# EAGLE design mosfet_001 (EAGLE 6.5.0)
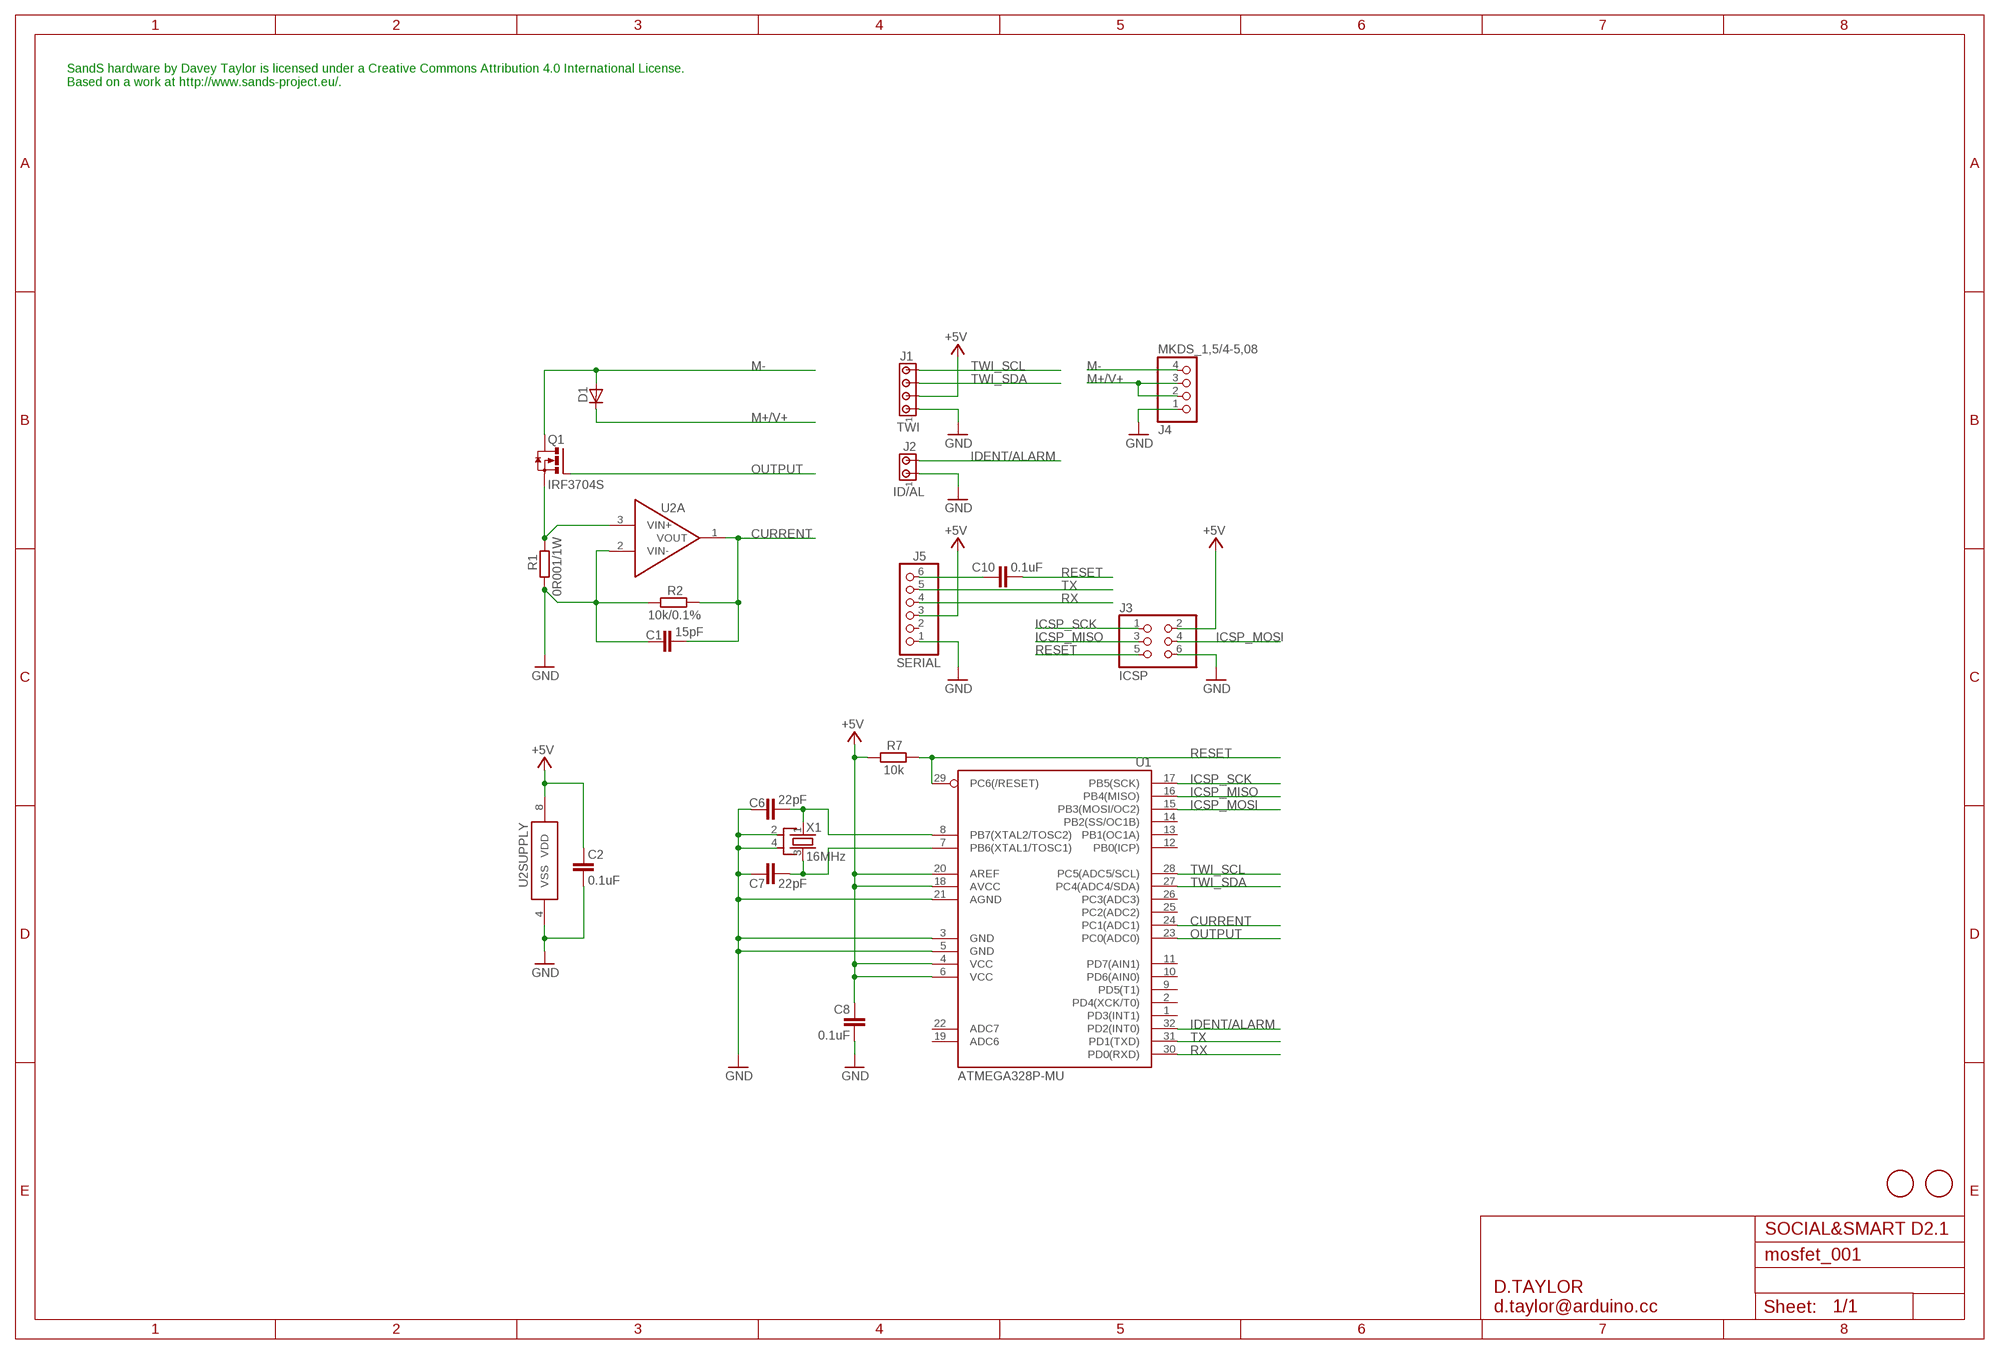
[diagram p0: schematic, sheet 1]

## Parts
C1  15pF  C-EUC0603  [C0603]
C2  0.1uF  C-EUC0603  [C0603]
C6  22pF  C-EUC0603  [C0603]
C7  22pF  C-EUC0603  [C0603]
C8  0.1uF  C-EUC0603  [C0603]
C10  0.1uF  C-EUC0603  [C0603]
D1  DIODE-SMB  [SMB]
J1  TWI  MTA04-100  [10X04MTA]
J2  ID/AL  MTA02-100  [10X02MTA]
J3  ICSP  PINHD-2X3  [2X03]
J4  MKDS_1,5/4-5,08  [MKDS1,5/4-5,08]
J5  SERIAL  PINHD-1X6  [1X06]
Q1  IRF3704S  [D2PACK]
R1  0R001/1W  R-EU_R2512  [R2512]
R2  10k/0.1%  R-EU_R0603  [R0603]
R7  10k  R-EU_R0603  [R0603]
U1  ATMEGA328P-MU  [MLF32-M1-A]
U2  LTC6081  [MSOP08]
U$5  FIDUCIALMOUNT  [FIDUCIA-MOUNT]
U$6  FIDUCIALMOUNT  [FIDUCIA-MOUNT]
X1  16MHz  CRYSTAL-KX7  [XTAL-3.2-2.5]

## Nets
+5V: C2.1 C8.1 J1.2 J3.2 J5.3 R7.1 U1.4(VCC) U1.6(VCC) U1.18(AVCC) U1.20(AREF) U2.8(SUPPLY:VDD)
CURRENT: C1.2 R2.2 U1.24(PC1(ADC1)) U2.1(A:VOUT)
GND: C1.1 C2.2 C6.1 C7.1 C8.2 J1.1 J2.1 J3.6 J4.1 J5.1 R1.1 R2.1 U1.3(GND) U1.5(GND) U1.21(AGND) U2.2(A:VIN-) U2.4(SUPPLY:VSS) X1.2(SH1) X1.4(SH2)
ICSP_MISO: J3.3 U1.16(PB4(MISO))
ICSP_MOSI: J3.4 U1.15(PB3(MOSI/OC2))
ICSP_SCK: J3.1 U1.17(PB5(SCK))
IDENT/ALARM: J2.2 U1.32(PD2(INT0))
M+/V+: D1.C J4.2 J4.3
M-: D1.A J4.4 Q1.2(D)
N$1: Q1.3(S) R1.2 U2.3(A:VIN+)
N$6: C6.2 U1.8(PB7(XTAL2/TOSC2)) X1.1(X1)
N$7: C7.2 U1.7(PB6(XTAL1/TOSC1)) X1.3(X2)
N$9: C10.1 J5.6
OUTPUT: Q1.1(G) U1.23(PC0(ADC0))
RESET: C10.2 J3.5 R7.2 U1.29(PC6(/RESET))
RX: J5.4 U1.30(PD0(RXD))
TWI_SCL: J1.4 U1.28(PC5(ADC5/SCL))
TWI_SDA: J1.3 U1.27(PC4(ADC4/SDA))
TX: J5.5 U1.31(PD1(TXD))
Unconnected: J5.2 U1.1(PD3(INT1)) U1.2(PD4(XCK/T0)) U1.9(PD5(T1)) U1.10(PD6(AIN0)) U1.11(PD7(AIN1)) U1.12(PB0(ICP)) U1.13(PB1(OC1A)) U1.14(PB2(SS/OC1B)) U1.19(ADC6) U1.22(ADC7) U1.25(PC2(ADC2)) U1.26(PC3(ADC3)) U2.5(B:VIN+) U2.6(B:VIN-) U2.7(B:VOUT)

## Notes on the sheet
- SandS hardware by Davey Taylor is licensed under a Creative Commons Attribution 4.0 International License.
  Based on a work at http://www.sands-project.eu/.
- SOCIAL&SMART D2.1
- D.TAYLOR
  d.taylor@arduino.cc

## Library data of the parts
C1 C2 C6-C8 C10 = rcl:C-EU: CAPACITOR, European symbol
D1 = diode:DIODE-: DIODE
J1 = con-amp:MTA04-100: AMP connector
J2 = con-amp:MTA02-100: AMP connector
J3 = pinhead:PINHD-2X3: PIN HEADER
J4 = d_taylor:MKDS_1,5/4-5,08
J5 = pinhead:PINHD-1X6: PIN HEADER
Q1 = transistor-power:IRF3704: SMPS MOSFET HEXFET® Power MOSFET Source: http://www.irf.com/product-info/datasheets/data/irf3704.pdf
R1 R2 R7 = rcl:R-EU_: RESISTOR, European symbol
U1 = d_taylor:ATMEGA*: MICROCONTROLLER 8 Kbytes FLASH 1 kbytes SRAM 512 bytes EEPROM USART 6-channel 10 bit ADC 2-channel 8 bit ADC Source: avr.lbr
U2 = d_taylor:LTC6081
U$5 U$6 = SmartPrj:FIDUCIALMOUNT
X1 = d_taylor:CRYSTAL-KX7

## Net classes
1 PWR: width 0.406 mm, clearance 0.254 mm

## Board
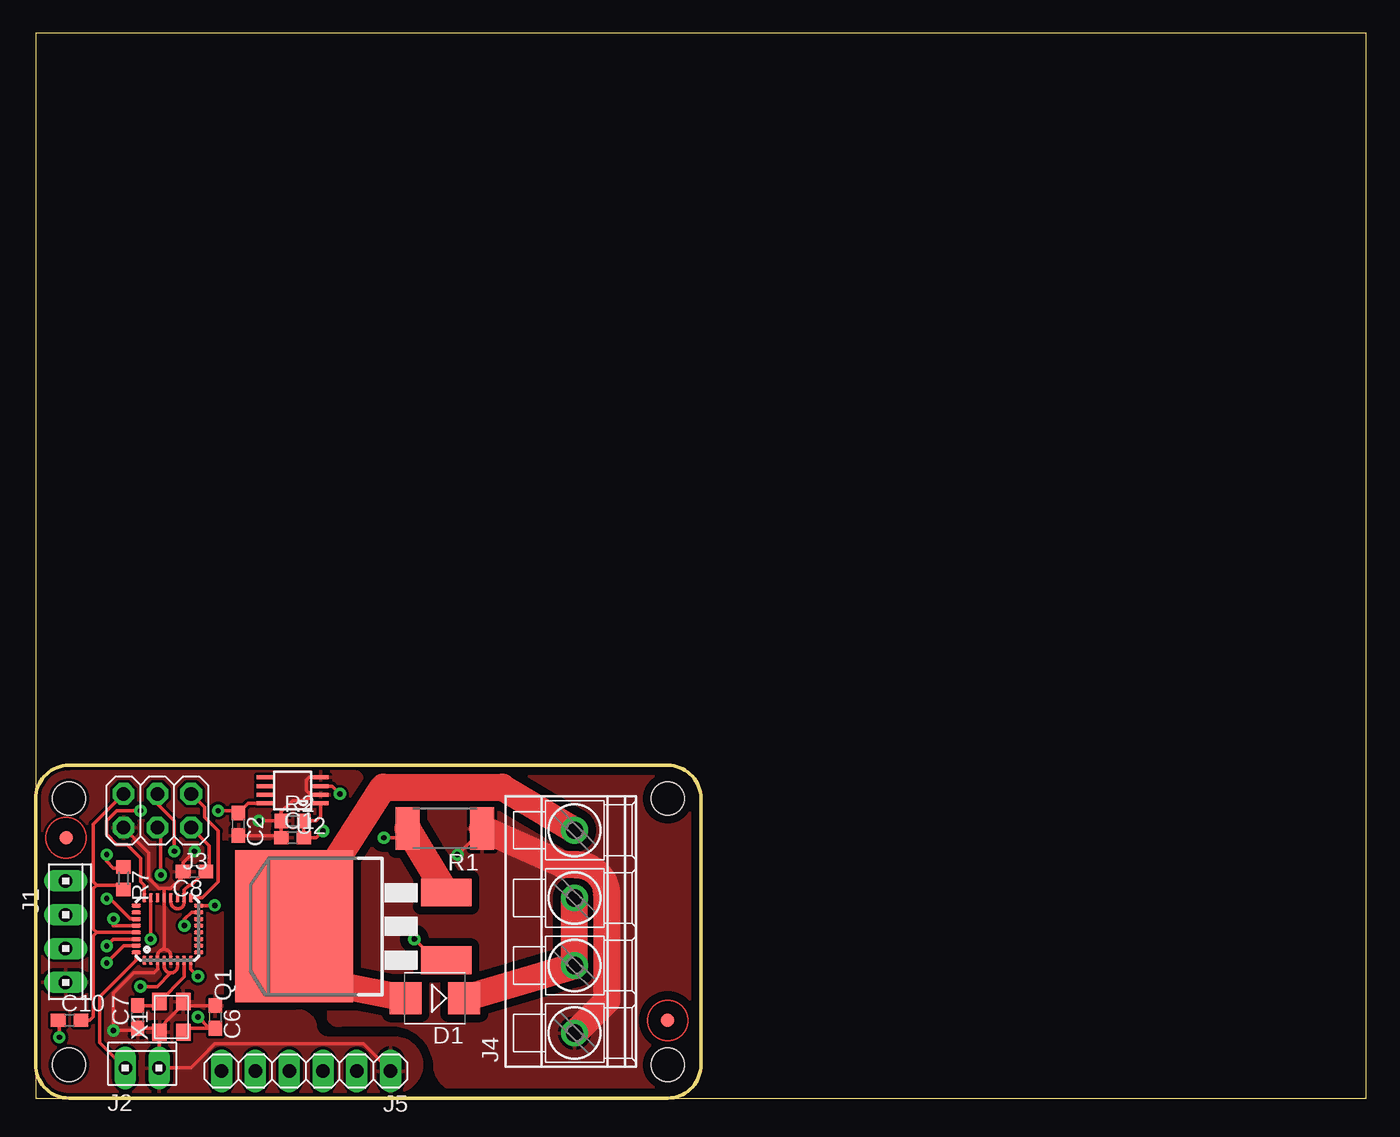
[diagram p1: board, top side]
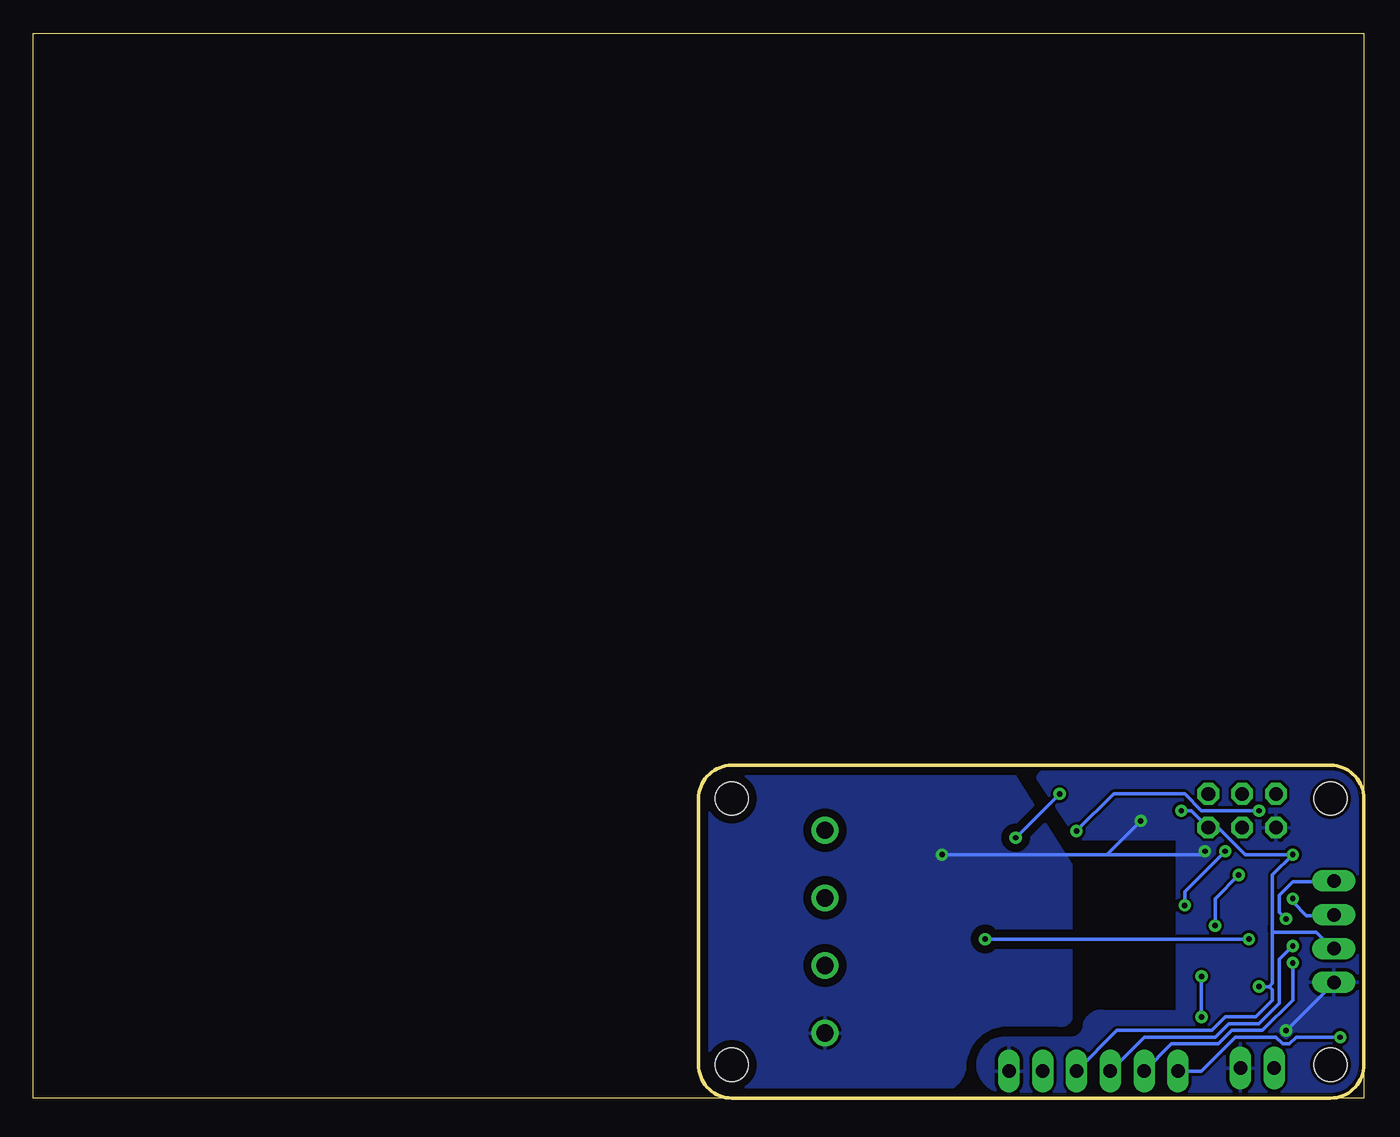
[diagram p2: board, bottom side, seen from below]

Size 100 x 80 mm. Coordinates in mm from the lower left corner, seen from the top.
Outline: 0,0 100,0 100,80 0,80 0,0
Outline: 2.5,0 47.5,0 arc90 50,2.5 50,22.5 arc90 47.5,25 2.5,25 arc90 0,22.5 0,2.5 arc90 2.5,0
Copper layers (1*16): Top 0.035mm / dielectric 1.5mm / Bottom 0.035mm
Design rules "smartprj-mini *": minimum track width 8mil, minimum drill 16mil, track to track 8mil, track to pad 8mil, pad to pad 0.200659375mm, via to via 8mil, smd to smd 4mil, copper to edge 10mil, drill to drill 8mil, minimum pad ring 12mil, minimum via ring 10mil, stop-mask expansion 2mil, vias tented up to drill 20mil, thermal gap 10mil
Holes 2.5 mm at 2.5,22.5 2.5,2.5 47.5,2.5 47.5,22.5

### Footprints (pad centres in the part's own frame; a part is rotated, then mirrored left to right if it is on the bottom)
C0603 = smd 1.1 x 1: 1 -0.85,0; 2 0.85,0
SMB = smd 2.4 x 2.4: A 2.2,0; C -2.2,0
10X04MTA = drill 1.016 long: 1 3.81,0; 2 1.27,0; 3 -1.27,0; 4 -3.81,0
10X02MTA = drill 1.016 long: 1 1.27,0; 2 -1.27,0
2X03 = drill 1.016 octagon: 1 -2.54,-1.27; 2 -2.54,1.27; 3 0,-1.27; 4 0,1.27; 5 2.54,-1.27; 6 2.54,1.27
MKDS1,5/4-5,08 = drill 1.3 pad 2: 1 -7.62,0; 2 -2.54,0; 3 2.54,0; 4 7.62,0
1X06 = drill 1.016 long: 1 -6.35,0; 2 -3.81,0; 3 -1.27,0; 4 1.27,0; 5 3.81,0; 6 6.35,0
D2PACK = smd 2.083 x 3.81: 1 -2.54,-8.89; 3 2.54,-8.89 | smd 11.43 x 8.89: 2 0,2.54
R2512 = smd 1.8 x 3.2: 1 -2.8,0; 2 2.8,0
R0603 = smd 1 x 1.1: 1 -0.85,0; 2 0.85,0
MLF32-M1-A = smd 0.7 x 0.3: 1 -2.35,1.75; 2 -2.35,1.25; 3 -2.35,0.75; 4 -2.35,0.25; 5 -2.35,-0.25; 6 -2.35,-0.75; 7 -2.35,-1.25; 8 -2.35,-1.75; 17 2.35,-1.75; 18 2.35,-1.25; 19 2.35,-0.75; 20 2.35,-0.25; 21 2.35,0.25; 22 2.35,0.75; 23 2.35,1.25; 24 2.35,1.75 | smd 0.3 x 0.7: 9 -1.75,-2.35; 10 -1.25,-2.35; 11 -0.75,-2.35; 12 -0.25,-2.35; 13 0.25,-2.35; 14 0.75,-2.35; 15 1.25,-2.35; 16 1.75,-2.35; 25 1.75,2.35; 26 1.25,2.35; 27 0.75,2.35; 28 0.25,2.35; 29 -0.25,2.35; 30 -0.75,2.35; 31 -1.25,2.35; 32 -1.75,2.35
MSOP08 = smd 0.3 x 1.2: 1 -0.976,-2.113; 2 -0.326,-2.113; 3 0.324,-2.113; 4 0.974,-2.113; 5 0.974,2.112; 6 0.324,2.112; 7 -0.326,2.112; 8 -0.976,2.112
FIDUCIA-MOUNT = smd 1.016 x 1.016: P$1 0,0
XTAL-3.2-2.5 = smd 1.3 x 1.1: 1 -1.15,-0.9; 2 1.15,-0.9; 3 1.15,0.9; 4 -1.15,0.9

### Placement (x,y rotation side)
C1  19.3,19.56 0 top
C2  15.24,20.57 270 top
C6  13.5,6.1 270 top
C7  7.66,6.1 90 top
C8  11.94,17.02 180 top
C10  2.54,5.84 0 top
D1  30,7.5 180 top
J1  2.25,12.5 270 top
J2  8,2.25 0 top
J3  9.14,21.59 180 top
J4  40.5,12.5 90 top
J5  20.32,2.03 180 top
Q1  21.96,12.9 90 top
R1  30.75,20.25 180 top
R2  19.3,20.83 0 top
R7  6.6,16.51 270 top
U1  9.91,12.7 90 top
U2  19.3,23.11 90 top
U$5  2.29,19.56 0 top
U$6  47.5,5.84 0 top
X1  10.2,6.1 90 top

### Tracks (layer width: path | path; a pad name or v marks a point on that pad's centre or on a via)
+5V  (via drill 0.41)
  Top 0.254: 11.18,15.32 U1.18 | 11.18,15.05 U1.18 | U1.4 9.66,9.9 arc90 10.16,9.4 | 10.16,9.4 arc90 10.66,9.89 U1.6 | 10.16,9.4 9.14,8.38 v7.87,8.38 | U1.18 11.16,15.64 11.52,16 11.68,16 12.7,17.02 C8.1 13.04,17.27 13.04,18.96 J3.2 | U1.18 11.16,14.71 arc-90 10.67,14.22 arc-90 10.16,14.74 U1.20 | U2.8 15.95,22.14 C2.1 15.07,21.59 v13.72,21.59 | v5.33,18.29 5.33,17.78 5.84,17.27 6.52,17.27 R7.1
  Bottom 0.254: 6.86,15.75 6.86,15.49 | 6.86,15.49 6.86,12.95 | 6.86,12.95 6.86,12.45 | 6.86,12.45 3.56,12.45 2.25,11.18 J1.2 | 6.86,12.45 6.86,12.95 | 6.86,12.95 6.86,8.64 7.11,8.38 | 7.11,8.38 6.86,8.13 6.86,7.37 7.37,6.86 8.13,6.1 10.41,6.1 11.43,5.08 18.54,5.08 J5.3 | 6.86,15.75 6.86,16.76 v5.33,18.29 8.89,18.29 10.92,20.32 J3.2 12.95,21.59 v13.72,21.59 | v7.87,8.38 7.11,8.38 | 6.86,15.75 6.86,15.49
CURRENT  (via drill 0.41)
  Top 0.254: U2.1 21.42,21.16 21.08,20.83 R2.2 C1.2 21.08,19.56 v21.59,20.07 | U1.24 8.16,15.97 7.87,16.26 7.87,18.03 6.86,19.05 6.1,19.05 5.33,19.81 5.33,20.83 6.1,21.59 v7.87,21.59
  Bottom 0.254: v7.87,21.59 12.19,21.59 13.46,22.86 18.8,22.86 v21.59,20.07
GND  (via drill 0.41)
  Top 0.254: 10.16,10.16 U1.5 10.16,10.68 arc90 9.66,11.18 | 9.14,10.35 U1.3 | 9.66,11.18 9.65,11.18 U1.21 9.65,15.75 | 9.14,10.35 U1.3 | 9.14,10.35 9.14,10.66 arc-90 9.66,11.18 | 13.41,6.95 C6.1 11.4,6.95 X1.2 11.1,7.04 10.16,6.1 9.3,5.24 X1.4 | J3.6 8.5,18.42 8.5,16.5 9.25,15.75 9.65,15.75 | 9.65,15.75 10.16,15.75 10.92,16.51 10.92,16.85 C8.2 11.09,17.69 v11.94,18.54 | R1.1 33.5,20.3 33.5,20.09 v31.7,18.29 | X1.4 9,5.25 C7.1 7.49,5.08 v5.84,5.08 5.84,7.87 7.37,9.4 8.89,9.4 9.16,9.66 U1.3 | X1.4 9.27,4.92 J2.1 9.3,2.29 9.91,2.29 11.68,2.29 12.45,3.05 13.46,4.06 24.64,4.06 J5.1 | U2.4 20.53,24.09 20.32,23.88 20.32,23.11 20.65,22.79 U2.2 20.76,22.79 20.32,22.35 19.3,22.35 18.45,21.5 R2.1 | R2.1 C1.1 18.29,19.72 C2.2 | R2.1 v16.76,20.83
  Top 2.032: J4.1 42.93,7.31 42.93,8 42.93,15.24 arc90 40.64,17.53 39.62,17.53 R1.1
  Bottom 0.254: v31.7,18.29 19.3,18.29 | 19.3,18.29 12.19,18.29 v11.94,18.54 | 2.25,8.64 5.3,5.59 v5.84,5.08 | v16.76,20.83 19.3,18.29
  pour Top: 0.5,22.5 arc-90 2.5,24.5 24,24.5 arc-90 24.5,24 21.5,19.5 14,19.5 14,6.5 19.5,6.5 arc-90 21,5.5 arc90 22,4.5 27,4.5 arc-90 29,2.5 arc-90 27,0.5 2.5,0.5 arc-90 0.5,2.5
  pour Top (isolate 0.61): 26.5,24.5 22,16 22,6 arc90 23,5.5 26.5,5.5 arc-90 30,2.5 arc90 32,0.5 47.5,0.5 arc90 49.5,2.5 49.5,22.5 arc90 47.5,24.5
  pour Bottom: 0.5,22.5 arc-90 2.5,24.5 24,24.5 arc-90 24.5,24 21.5,19.5 14,19.5 14,6.5 19.5,6.5 arc-90 21,5.5 arc90 22,4.5 27,4.5 arc-90 29,2.5 arc-90 27,0.5 2.5,0.5 arc-90 0.5,2.5
  pour Bottom (isolate 0.61): 26.5,24.5 22,17.5 22,6 arc90 23,5.5 26.5,5.5 arc-90 30,2.5 arc90 32,0.5 47.5,0.5 arc90 49.5,2.5 49.5,22.5 arc90 47.5,24.5
ICSP_MISO  (via drill 0.41)
  Top 0.254: J3.3 9.14,22.1 10.41,20.83 10.41,19.56 v10.41,18.54 | v13.46,14.48 13.72,14.45 U1.16
  Bottom 0.254: v10.41,18.54 13.46,15.49 v13.46,14.48
ICSP_MOSI  (via drill 0.41)
  Top 0.254: J3.4 9.4,20.07 v9.4,16.76 | U1.15 11.7,13.95 11.18,13.42 v11.18,12.95
  Bottom 0.254: v9.4,16.76 11.18,14.99 v11.18,12.95
ICSP_SCK
  Top 0.254: U1.17 12.51,15.05 13.72,16.26 13.72,20.07 12.7,21.08 12.7,21.84 J3.1
IDENT/ALARM
  Top 0.254: J2.2 4.83,4.16 4.83,7.61 7.56,10.34 U1.32
M+/V+
  Top 2.032: J4.3 J4.2 D1.C
M-
  Top 2.032: D1.A 22.44,8.54 Q1.2 26.13,23.37 35.05,23.37 J4.4
N$1  (via drill 0.41)
  Top 0.254: U2.3 22.28,23.44 v22.86,22.86 | v26.16,19.56 27.27,19.56 R1.2
  Top 2.032: Q1.3 R1.2
  Bottom 0.254: v26.16,19.56 v22.86,22.86
N$6  (via drill 0.41)
  Top 0.254: X1.1 11.4,5.25 C6.2 13.04,5.25 v12.19,6.1 | v12.19,9.14 11.66,9.68 U1.8
  Bottom 0.254: v12.19,6.1 v12.19,9.14
N$7
  Top 0.254: 7.66,7.11 C7.2 9,6.95 X1.3 11.16,9.1 U1.7
N$9  (via drill 0.41)
  Top 0.254: v1.78,4.57 1.78,5.84 C10.1
  Bottom 0.254: J5.6 12.19,2.03 9.65,4.57 6.6,4.57 6.1,4.06 5.59,4.06 5.08,4.57 v1.78,4.57
OUTPUT  (via drill 0.41)
  Top 0.254: U1.23 8.66,11.96 v8.64,11.94 | Q1.1 30.04,10.36 v28.46,11.94
  Bottom 0.254: v8.64,11.94 v28.46,11.94
RESET
  Top 0.254: U1.29 5.84,12.45 4.57,12.45 | 4.57,12.45 4.32,12.7 4.32,15.75 4.57,16 | C10.2 4.06,5.84 4.32,6.1 4.32,12.19 4.57,12.45 | R7.2 6.6,16 4.57,16 | 4.57,16 4.32,16.26 4.32,19.56 4.32,20.57 J3.5
RX  (via drill 0.41)
  Top 0.254: U1.30 7.56,11.94 5.84,11.94 v5.33,11.43
  Bottom 0.254: v5.33,11.43 6.35,10.41 6.35,7.11 6.86,6.6 7.87,5.59 10.16,5.59 11.18,4.57 16.51,4.57 J5.4
TWI_SCL  (via drill 0.41)
  Top 0.254: U1.28 5.84,12.95 v5.84,13.46
  Bottom 0.254: v5.84,13.46 6.35,13.97 6.35,15.24 5.33,16.26 2.29,16.26 2.29,16.31 J1.4
TWI_SDA  (via drill 0.41)
  Top 0.254: v5.33,14.99 5.59,14.99 7.11,13.46 7.56,13.46 U1.27
  Bottom 0.254: J1.3 2.25,13.72 4.32,13.72 5.33,14.73 v5.33,14.99
TX  (via drill 0.41)
  Top 0.254: U1.31 6.6,11.45 v5.33,10.16
  Bottom 0.254: v5.33,10.16 5.33,7.37 7.62,5.08 9.91,5.08 10.92,4.06 14.48,4.06 J5.5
